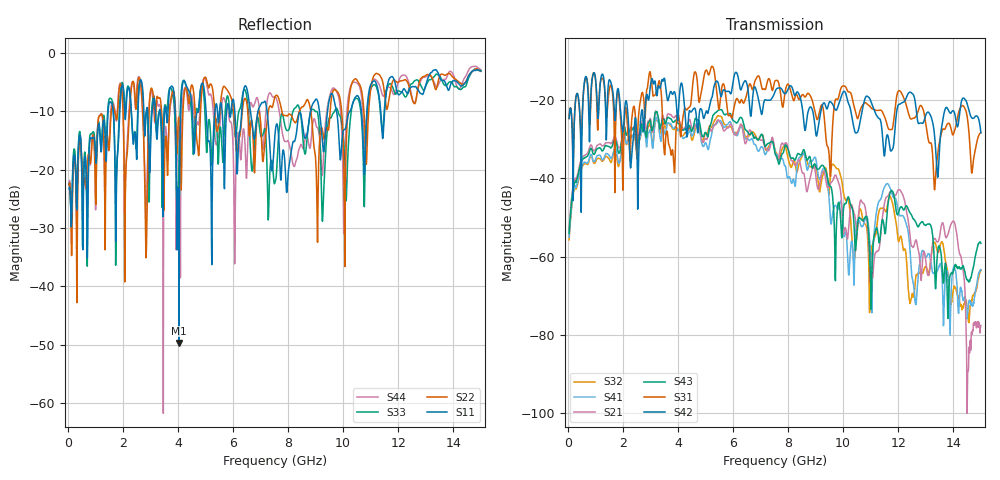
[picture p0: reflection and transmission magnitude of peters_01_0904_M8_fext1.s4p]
# MHZ S RI R 50.00
! FREQ  S11  S12  S13  S14
!  S21  S22  S23  S24
!  S31  S32  S33  S34
!  S41  S42  S43  S44
!  REAL  IMAG  REAL  IMAG  REAL  IMAG  REAL  IMAG
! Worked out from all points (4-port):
!   1496 points, 50 MHz to 15 GHz, reference 50 ohm
!   strongest paths, dB at 50 MHz, 3.79 GHz, 7.53 GHz, 11.27 GHz, 15 GHz:
!     S42: -24.7, -18.5, -17.8, -24.6, -28.4
!     S31: -24.8, -32.9, -15.1, -22.7, -28.3
!     S43: -54.1, -25.4, -33.8, -54.5, -56.6
!     S21: -53.3, -24.2, -33.4, -58.5, -77.5
!     S41: -55.1, -26.9, -33.2, -46.4, -63.3
!     S32: -55.7, -27.2, -32.9, -49.5, -63.6
!   lowest |S11| = -49.7 dB at 4.04 GHz (marker M1), VSWR 1.01, Z = 50.3 - j0.14 ohm
!   |S11| at or under -10 dB: start of sweep to 1.465 GHz; 7.237 GHz to 8.816 GHz (1.579 GHz wide, 19.7 % of centre); 9.757 GHz to 10.25 GHz (489 MHz wide, 4.89 % of centre)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
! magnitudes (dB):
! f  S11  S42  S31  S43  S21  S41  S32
! 50 MHz  -23.3  -24.7  -24.8  -54.1  -53.3  -55.1  -55.7
! 4.04 GHz  -49.7  -20.4  -24.6  -26.0  -25.4  -27.4  -27.6
! 11.04 GHz  -5.1  -21.1  -22.3  -65.0  -64.1  -74.3  -57.3
! 11.6 GHz  -5.6  -28.9  -26.5  -48.3  -44.7  -41.4  -47.1
! 12.61 GHz  -5.7  -20.3  -24.5  -50.9  -56.2  -71.6  -67.1
! 14 GHz  -4.7  -22.8  -28.8  -63.7  -50.9  -63.0  -68.3
! 15 GHz  -3.1  -28.4  -28.3  -56.6  -77.5  -63.3  -63.6
